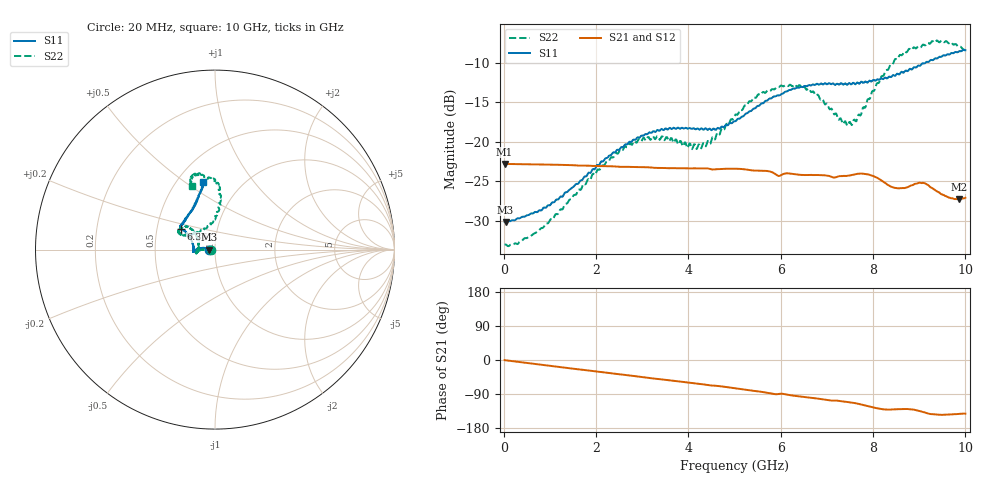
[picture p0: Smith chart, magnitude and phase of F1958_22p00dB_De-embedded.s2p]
! Integrated Device Technology
! Corporate Headquarters
! 6024 Silver Creek Valley Road
! San Jose, CA 95138  USA
! Phone:  1-408-284-8200
! Toll Free:  1-800-223-1366
! Webpage:  http://www.idt.com/
! Timing and RF Division
! 515 Groton Road, Suite 102
! Westford, MA 01886-6024
! Device:  F1958
! Description: 7-bit 0.25 dB Digital Step Attenuator
! Frequency:  0.001 -  6.000 GHz
! Package:  4x4 mm Thin QFN Plastic Package: 24 pin
! Ports:  2 RF, 12 DC
!  Pin  1  = D0
!  Pin  2  = VDD
!  Pin  3  = VMODE
!  Pin  4  = GND
!  Pin  5  = RF1  =  Port 1
!  Pin  6  = GND
!  Pin  7  = GND
!  Pin  8  = GND
!  Pin  9  = GND
!  Pin 10  = GND
!  Pin 11  = GND
!  Pin 12  = GND
!  Pin 13  = GND
!  Pin 14  = RF2  =  Port 2
!  Pin 15  = GND
!  Pin 16  = LE
!  Pin 17  = CLK
!  Pin 18  = DATA
!  Pin 19  = D6
!  Pin 20  = D5
!  Pin 21  = D4
!  Pin 22  = D3
!  Pin 23  = D2
!  Pin 24  = D1
! State:  88
! Atten State:  22.00 dB
! Voltage:  +3.30 Volts
! Current:  0.257 mA
! Data:  The device was measured on a F1958 evaluation board which has
!  individual transmission lines to the RF pins.  Data was collected
!  using a calibrated network analyzer.  The evaluation board was
!  de-embedded using Automatic Fixture Removal (AFR).
!  The reference plane is the edge of the package pin.
! Misc:
!  Action Tracker AT0419
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# GHz S dB R 50
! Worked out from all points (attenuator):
!   500 points, 20 MHz to 10 GHz, reference 50 ohm
!   highest |S21| = -22.81 dB at 20 MHz (marker M1); lowest = -27.3 dB at 9.86 GHz (marker M2)
!   lowest |S11| = -30.2 dB at 40 MHz (marker M3), VSWR 1.06, Z = 47 - j0.0431 ohm
!   |S11| at or under -10 dB: start of sweep to 9.133 GHz
!   |S22| runs from -33.2 to -7.2 dB; largest |S21 - S12| = 0.00033
!   S11 on the Smith chart (normalised r, x): 20 MHz: 0.94, -0.00; 6.36 GHz: 0.67, +0.16; 10 GHz: 0.67, +0.59
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0.02  -30.14 -178.9  -22.81 -0.4  -22.81 -0.3  -33.06 -178.3
0.04  -30.17 -179.2  -22.81 -0.7  -22.81 -0.6  -33.01 -177.5
0.32  -29.70 175.2  -22.84 -5.0  -22.84 -5.0  -32.86 177.4
0.84  -28.55 171.1  -22.89 -12.9  -22.88 -12.8  -30.93 178.5
1.7  -24.86 171.2  -23.03 -25.7  -23.02 -25.6  -25.68 177.7
2.6  -20.59 177.2  -23.18 -39.0  -23.16 -39.0  -20.83 -176.9
3.36  -18.60 -175.3  -23.32 -50.3  -23.32 -50.5  -19.58 -168.3
4.26  -18.40 -179.6  -23.37 -63.3  -23.38 -63.4  -20.70 169.5
5.02  -17.40 161.2  -23.42 -74.7  -23.43 -74.8  -16.55 140.1
5.58  -15.15 150.9  -23.68 -83.9  -23.69 -83.9  -13.97 140.3
6.36  -13.13 148.4  -24.15 -95.4  -24.16 -95.3  -13.06 153.7
6.68  -12.79 146.9  -24.21 -99.7  -24.23 -99.6  -13.68 154.9
7.32  -12.61 141.6  -24.36 -109.0  -24.37 -108.8  -17.34 134.9
7.5  -12.61 138.5  -24.27 -111.5  -24.27 -111.5  -17.49 117.1
7.68  -12.57 135.6  -24.05 -115.5  -24.06 -115.5  -16.60 99.6
7.92  -12.26 129.3  -24.19 -122.8  -24.17 -122.9  -14.61 89.0
8.34  -11.76 119.3  -25.52 -130.9  -25.53 -131.0  -10.73 83.6
8.68  -11.13 112.5  -25.87 -129.4  -25.87 -129.3  -8.56 87.9
9.04  -10.26 107.1  -25.23 -135.6  -25.22 -135.7  -8.01 95.5
9.26  -9.63 105.0  -25.81 -142.7  -25.81 -142.6  -7.38 100.5
9.86  -8.55 100.0  -27.28 -142.0  -27.32 -142.1  -7.95 109.1
10  -8.41 100.0  -27.09 -141.7  -27.15 -141.5  -8.43 109.9
